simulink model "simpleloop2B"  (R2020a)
settings: Solver=ode45  StartTime=0.0  StopTime=10.0  RelTol=1e-3  EnableMultiTasking=on

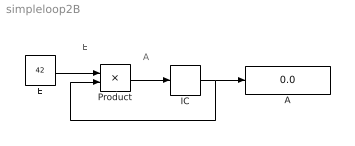
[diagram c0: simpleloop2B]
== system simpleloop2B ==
  note: A
  note: E
  note: .
  A : Display
  E : Constant  Value=42
  IC : InitialCondition
  Product : Product  Inputs=*/  SaturateOnIntegerOverflow=on
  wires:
  E/1 -> Product/1
  Product/1 -> IC/1
  IC/1 -> A/1, Product/2
